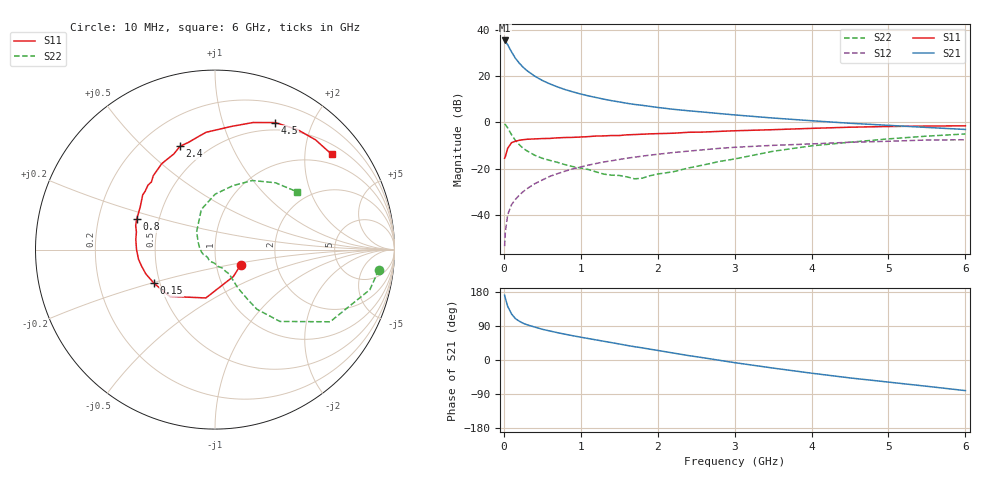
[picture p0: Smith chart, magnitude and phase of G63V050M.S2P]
! SIEMENS Small Signal Semiconductors
! BFG193
! Si NPN RF Bipolar Junction Transistor in SOT223
! VCE = 3 V  IC = 50 mA
! Common Emitter S-Parameters:  August  1996
# GHz  S  MA  R  50
!  f  S11  S21  S12  S22
! GHz  MAG  ANG  MAG  ANG  MAG  ANG  MAG  ANG
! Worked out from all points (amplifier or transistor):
!   36 points, 10 MHz to 6 GHz, reference 50 ohm
!   highest |S21| = 35.4 dB at 10 MHz (marker M1)
!   |S21| within 3 dB of that: start of sweep to 68.39 MHz
!   unconditionally stable (mu >= 1): 411.9 MHz to 2.348 GHz
!   at 250 MHz: K = 0.92, MSG = 26.9 dB, |S12| = -30.0 dB
!   at 1.4 GHz: K = 1.04, MAG = 11.7 dB, |S12| = -16.6 dB
!   at 6 GHz: K = 0.90, MSG = 2.2 dB, |S12| = -7.6 dB
!   S11 on the Smith chart (normalised r, x): 10 MHz: 1.31, -0.23; 150 MHz: 0.46, -0.21; 800 MHz: 0.37, +0.16; 2.4 GHz: 0.36, +0.65; 4.5 GHz: 0.41, +1.50; 6 GHz: 0.73, +2.62
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0.01  0.1667 -30.6  58.75 170.8  0.0021 90.3  0.919 -7.1
0.02  0.1816 -55.8  56.46 162.8  0.0043 80.6  0.8913 -14.5
0.05  0.2742 -100.7  47.38 141.5  0.0101 71.7  0.7569 -32.1
0.1  0.3629 -134.1  33.25 121.5  0.0166 65.1  0.5395 -47.9
0.15  0.3883 -151.1  24.26 109.3  0.0215 66.0  0.4061 -54.9
0.2  0.4087 -160.7  19.07 102.5  0.0265 67.6  0.3295 -56.8
0.25  0.42 -167.7  15.53 97.0  0.0316 68.0  0.2741 -58.3
0.3  0.4295 -172.8  13.12 93.1  0.0366 69.4  0.242 -59.2
0.4  0.4372 180.0  9.984 87.0  0.0469 69.4  0.1944 -59.6
0.5  0.4448 172.7  8.027 81.1  0.0566 68.0  0.1667 -59.7
0.6  0.4486 167.4  6.737 76.5  0.068 67.4  0.15 -61.0
0.7  0.4618 163.1  5.801 72.0  0.0779 65.8  0.1357 -63.8
0.8  0.4689 158.5  5.071 67.9  0.0882 64.1  0.1208 -66.5
1.1  0.4903 146.8  3.723 56.6  0.1187 58.8  0.0951 -80.1
1.3  0.5074 139.9  3.162 49.4  0.1388 54.5  0.0758 -92.2
1.6  0.5359 130.0  2.575 38.5  0.1672 47.7  0.0661 -121.4
2.2  0.58 113.3  1.913 18.5  0.2218 34.0  0.0852 175.8
2.4  0.608 108.7  1.775 11.7  0.2381 29.7  0.1029 155.9
3.5  0.6924 82.4  1.236 -21.3  0.3174 2.4  0.2365 108.8
4.5  0.7832 64.6  0.953 -47.3  0.3704 -17.6  0.3712 74.1
5.5  0.8292 47.6  0.774 -69.4  0.4142 -40.9  0.5024 47.8
6  0.8389 39.3  0.7 -80.8  0.4187 -54.2  0.5596 35.1
